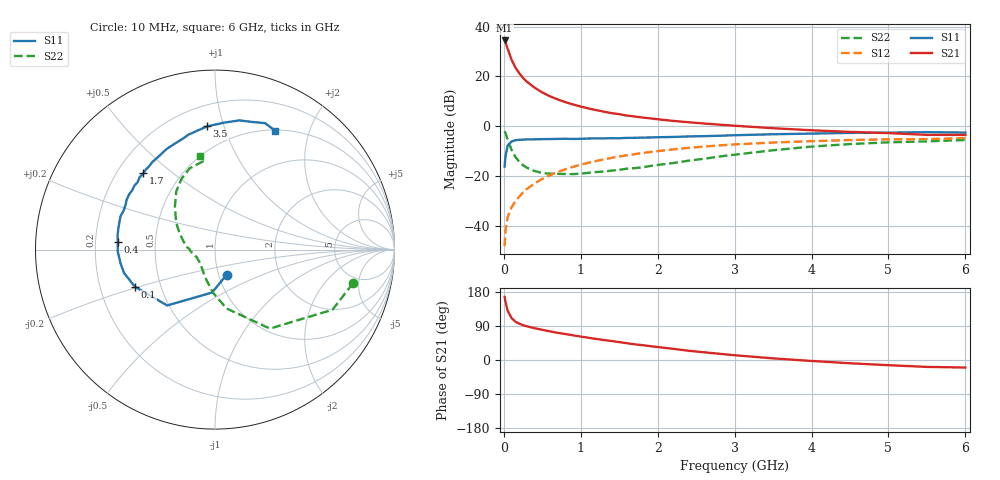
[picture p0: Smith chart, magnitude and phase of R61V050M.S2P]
! SIEMENS Small Signal Semiconductors
! BFR193
! Si NPN RF Bipolar Junction Transistor in SOT23
! VCE = 1 V  IC = 50 mA
! Common Emitter S-Parameters:  May  1996
# GHz  S  MA  R  50
!  f  S11  S21  S12  S22
! GHz  MAG  ANG  MAG  ANG  MAG  ANG  MAG  ANG
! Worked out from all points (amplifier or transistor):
!   36 points, 10 MHz to 6 GHz, reference 50 ohm
!   highest |S21| = 34.4 dB at 10 MHz (marker M1)
!   |S21| within 3 dB of that: start of sweep to 46.18 MHz
!   unconditionally stable (mu >= 1): 231.5 MHz to 2.442 GHz
!   at 250 MHz: K = 1.01, MAG = 22.3 dB, |S12| = -26.6 dB
!   at 1.4 GHz: K = 1.05, MAG = 7.6 dB, |S12| = -12.7 dB
!   at 6 GHz: K = 1.00, MSG = 0.6 dB, |S12| = -4.8 dB
!   S11 on the Smith chart (normalised r, x): 10 MHz: 1.09, -0.31; 100 MHz: 0.36, -0.19; 400 MHz: 0.30, +0.04; 1.7 GHz: 0.31, +0.40; 3.5 GHz: 0.34, +0.88; 6 GHz: 0.51, +1.50
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0.01  0.1544 -64.9  52.53 166.7  0.0039 75.3  0.7912 -13.7
0.02  0.24 -94.0  49.18 154.5  0.0078 71.2  0.7356 -27.1
0.05  0.4097 -130.6  35.7 129.8  0.015 65.0  0.536 -55.2
0.1  0.4917 -155.1  21.65 110.7  0.0234 64.6  0.3348 -78.8
0.15  0.523 -165.5  15.12 101.4  0.0311 66.8  0.2417 -92.4
0.2  0.5319 -171.7  11.58 95.8  0.0384 69.8  0.1933 -101.1
0.25  0.5367 -176.1  9.279 91.9  0.0468 70.8  0.164 -109.4
0.3  0.5421 -178.8  7.784 88.8  0.0548 71.9  0.1464 -115.5
0.4  0.5437 175.3  5.929 84.0  0.0711 72.6  0.1258 -125.5
0.5  0.549 171.4  4.75 79.7  0.0874 72.5  0.1147 -134.2
0.6  0.5513 167.2  3.978 75.5  0.1038 71.5  0.111 -140.8
0.7  0.5548 163.5  3.438 71.7  0.1201 70.5  0.1101 -146.1
0.9  0.5537 157.1  2.723 65.1  0.153 67.7  0.1091 -155.9
1.1  0.5652 150.6  2.269 58.7  0.1846 64.7  0.1159 -162.1
1.4  0.5734 141.5  1.828 50.2  0.2309 59.7  0.128 -171.9
1.7  0.5831 133.2  1.562 41.4  0.274 54.7  0.1437 178.3
2.2  0.6071 120.8  1.276 29.5  0.3416 46.0  0.182 165.3
2.8  0.6421 106.6  1.073 16.5  0.4108 35.7  0.2456 148.6
3.5  0.6879 93.7  0.91 4.3  0.4693 23.9  0.3282 132.9
4.5  0.7325 79.3  0.767 -8.6  0.526 9.8  0.4372 115.2
5.5  0.7578 68.4  0.669 -18.2  0.5484 -3.3  0.4958 97.9
6  0.7425 63.2  0.668 -19.9  0.5777 -7.2  0.5273 99.1
